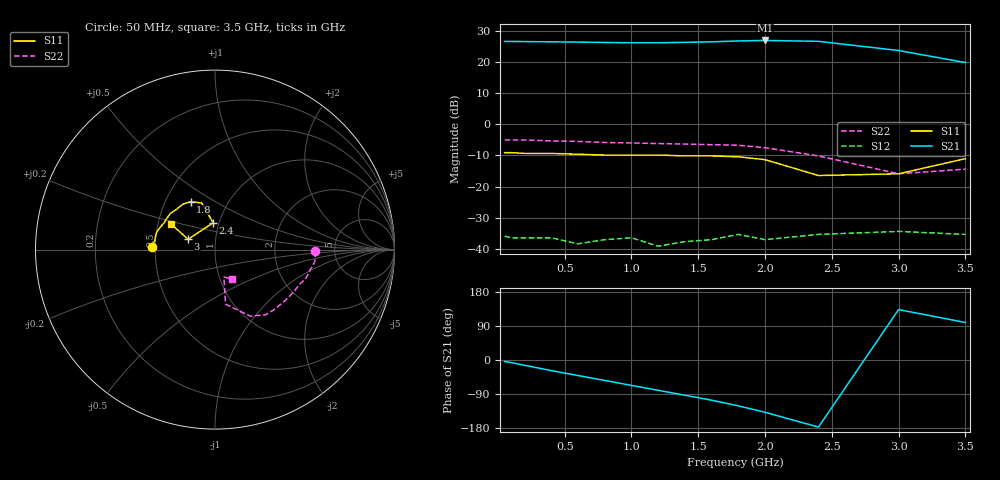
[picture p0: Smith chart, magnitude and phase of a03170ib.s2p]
!  INA-03170  S AND NOISE PARAMETERS
!  Id = 12 mA  LAST UPDATED 07-22-92
# ghz s ma r 50
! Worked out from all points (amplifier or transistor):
!   15 points, 50 MHz to 3.5 GHz, reference 50 ohm
!   highest |S21| = 26.9 dB at 2 GHz (marker M1)
!   |S21| within 3 dB of that: start of sweep to 2.953 GHz
!   unconditionally stable (mu >= 1): start of sweep to end of sweep
!   at 200 MHz: K = 1.30, MAG = 28.2 dB, |S12| = -36.5 dB
!   at 1.2 GHz: K = 1.79, MAG = 27.5 dB, |S12| = -39.2 dB
!   at 3.5 GHz: K = 2.71, MAG = 20.4 dB, |S12| = -35.4 dB
!   lowest NFmin = 1.60 dB at 10 MHz
!   S11 on the Smith chart (normalised r, x): 50 MHz: 0.48, +0.01; 1.8 GHz: 0.67, +0.39; 2.4 GHz: 0.94, +0.29; 3 GHz: 0.74, +0.09; 3.5 GHz: 0.59, +0.18
0.05  0.35 178.0  21.4 -4.0  0.016 9.0  0.56 -1.0
0.1  0.35 176.0  21.4 -7.0  0.015 6.0  0.56 -4.0
0.2  0.34 172.0  21.3 -14.0  0.015 -1.0  0.56 -7.0
0.4  0.34 164.0  21.1 -28.0  0.015 -5.0  0.54 -13.0
0.6  0.33 158.0  20.9 -41.0  0.012 2.0  0.53 -18.0
0.8  0.32 152.0  20.6 -54.0  0.014 5.0  0.51 -22.0
1  0.32 147.0  20.4 -67.0  0.015 4.0  0.5 -27.0
1.2  0.32 141.0  20.4 -80.0  0.011 13.0  0.49 -32.0
1.4  0.31 133.0  20.7 -93.0  0.013 25.0  0.48 -38.0
1.6  0.31 125.0  21.1 -106.0  0.014 28.0  0.47 -45.0
1.8  0.3 117.0  21.8 -121.0  0.017 30.0  0.46 -52.0
2  0.27 106.0  22.2 -138.0  0.014 33.0  0.42 -62.0
2.4  0.15 94.0  21.5 -177.0  0.017 23.0  0.31 -79.0
3  0.16 159.0  15.3 133.0  0.019 42.0  0.16 -72.0
3.5  0.28 150.0  9.8 99.0  0.017 28.0  0.19 -60.0
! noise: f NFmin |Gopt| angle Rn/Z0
0.01  1.6  0.44  0  0.49
0.1  1.6  0.44  3  0.49
0.5  1.7  0.42  17  0.48
1  2  0.36  35  0.47
2  3  0.21  81  0.42
